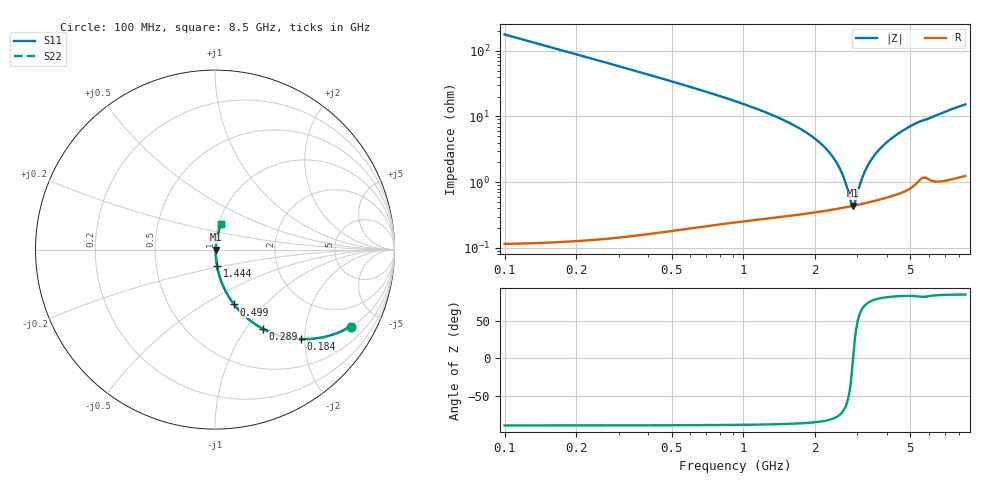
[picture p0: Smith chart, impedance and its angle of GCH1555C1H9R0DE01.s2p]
!Murata Part Number: GCH1555C1H9R0DE01
!These Parameters are Measured in Series Mode Connection
!Data Generated on Jun 19, 2026
!  o--ll--o
!Port1  Port2
!  o------o
!Operation Temp=25[degC], DC Bias Voltage=0[V]
!Freq. Start=100[MHz] Stop=9[GHz] 401[Steps]
# Hz S RI R 50
!Freq.(Hz) S11(Real) S11(Imag) S21(Real) S21(Imag) S12(Real) S12(Imag) S22(Real) S22(Imag)
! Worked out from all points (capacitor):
!   401 points, 100 MHz to 8.5 GHz, reference 50 ohm
!   read as one part in series: C = 9.01 pF near 142 MHz
!   lowest |Z| = 438 mohm at 2.872 GHz (marker M1)
!   series resonance near 2.879 GHz, so ESL is about 340 pH
!   S11 on the Smith chart (normalised r, x): 100 MHz: 1.00, -3.53; 184 MHz: 1.00, -1.91; 289 MHz: 1.00, -1.21; 499 MHz: 1.00, -0.69; 1.444 GHz: 1.01, -0.18; 8.5 GHz: 1.02, +0.30
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1e8  0.7571 -0.4285  0.2429 0.4285  0.2429 0.4285  0.7571 -0.4285
1.84e8  0.4779 -0.4989  0.5221 0.4989  0.5221 0.4989  0.4779 -0.4989
2.89e8  0.2685 -0.442  0.7315 0.442  0.7315 0.442  0.2685 -0.442
3.73e8  0.1789 -0.3816  0.8211 0.3816  0.8211 0.3816  0.1789 -0.3816
4.99e8  0.1065 -0.3058  0.8935 0.3058  0.8935 0.3058  0.1065 -0.3058
8.77e8  0.0343 -0.1755  0.9657 0.1755  0.9657 0.1755  0.0343 -0.1755
1.444e9  0.0111 -0.0898  0.9889 0.0898  0.9889 0.0898  0.0111 -0.0898
1.507e9  0.0101 -0.0835  0.9899 0.0835  0.9899 0.0835  0.0101 -0.0835
2.032e9  0.00535 -0.0429  0.9947 0.0429  0.9947 0.0429  0.00535 -0.0429
2.368e9  0.00439 -0.0237  0.9956 0.0237  0.9956 0.0237  0.00439 -0.0237
2.578e9  0.00421 -0.0133  0.9958 0.0133  0.9958 0.0133  0.00421 -0.0133
2.809e9  0.00429 -0.00296  0.9957 0.00296  0.9957 0.00296  0.00429 -0.00296
2.872e9  0.00436 -0.000281  0.9956 0.000281  0.9956 0.000281  0.00436 -0.000281
2.914e9  0.00441 0.00147  0.9956 -0.00147  0.9956 -0.00147  0.00441 0.00147
3.145e9  0.00479 0.0107  0.9952 -0.0107  0.9952 -0.0107  0.00479 0.0107
3.397e9  0.00539 0.02  0.9946 -0.02  0.9946 -0.02  0.00539 0.02
3.775e9  0.00659 0.0329  0.9934 -0.0329  0.9934 -0.0329  0.00659 0.0329
4.3e9  0.00876 0.0493  0.9912 -0.0493  0.9912 -0.0493  0.00876 0.0493
5.035e9  0.0131 0.0702  0.9869 -0.0702  0.9869 -0.0702  0.0131 0.0702
5.707e9  0.019 0.0847  0.981 -0.0847  0.981 -0.0847  0.019 0.0847
7.114e9  0.0244 0.1164  0.9756 -0.1164  0.9756 -0.1164  0.0244 0.1164
8.5e9  0.0341 0.145  0.9659 -0.145  0.9659 -0.145  0.0341 0.145
